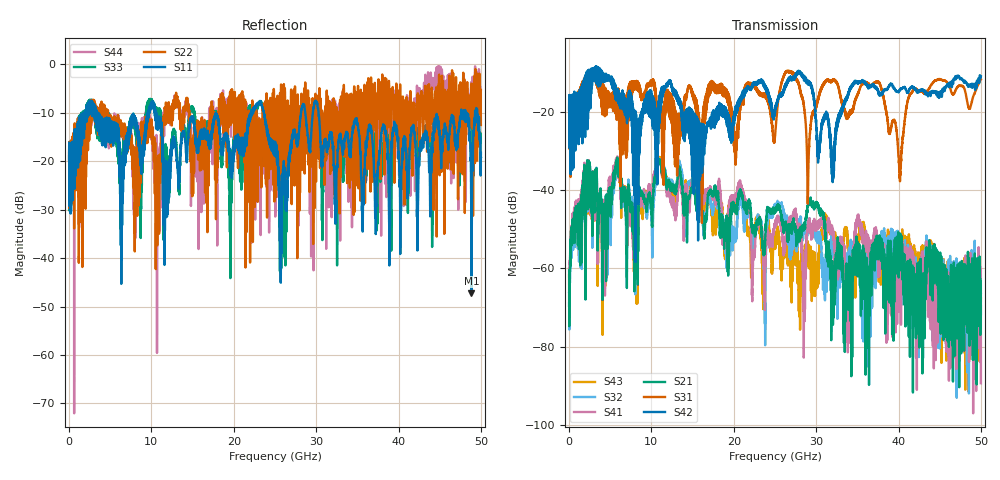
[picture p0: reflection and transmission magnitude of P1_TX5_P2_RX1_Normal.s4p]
!Keysight Technologies,N5225B,MY57041031,A.13.20.10
!Date: Friday, May 31, 2019 11:28:32
!Correction: S11(Full 4 Port(1,2,3,4))
!S12(Full 4 Port(1,2,3,4))
!S13(Full 4 Port(1,2,3,4))
!S14(Full 4 Port(1,2,3,4))
!S21(Full 4 Port(1,2,3,4))
!S22(Full 4 Port(1,2,3,4))
!S23(Full 4 Port(1,2,3,4))
!S24(Full 4 Port(1,2,3,4))
!S31(Full 4 Port(1,2,3,4))
!S32(Full 4 Port(1,2,3,4))
!S33(Full 4 Port(1,2,3,4))
!S34(Full 4 Port(1,2,3,4))
!S41(Full 4 Port(1,2,3,4))
!S42(Full 4 Port(1,2,3,4))
!S43(Full 4 Port(1,2,3,4))
!S44(Full 4 Port(1,2,3,4))
!S4P File: Measurements: <S11,S12,S13,S14>,
!<S21,S22,S23,S24>,
!<S31,S32,S33,S34>,
!<S41,S42,S43,S44>:
# Hz S  dB  R 50.0
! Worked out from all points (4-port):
!   5000 points, 10 MHz to 50 GHz, reference 50 ohm
!   strongest paths, dB at 10 MHz, 12.51 GHz, 25.01 GHz, 37.51 GHz, 50 GHz:
!     S42: -19.5, -14.3, -20.2, -14.6, -10.9
!     S31: -19.3, -23.1, -26.1, -12.2, -11.7
!     S21: -69.5, -38.9, -45.6, -55.1, -71.6
!     S41: -60.0, -42.5, -49.0, -56.1, -89.4
!     S32: -66.3, -37.4, -43.6, -53.9, -66.3
!     S43: -61.8, -40.2, -51.5, -57.7, -67.7
!   lowest |S11| = -47.3 dB at 48.86 GHz (marker M1), VSWR 1.01, Z = 50 - j0.434 ohm
!   |S11| at or under -10 dB: 3.502 GHz to 9.556 GHz (6.054 GHz wide, 92.7 % of centre); 10.5 GHz to 22.11 GHz (11.6 GHz wide, 71.2 % of centre); 30.29 GHz to 47.59 GHz (17.3 GHz wide, 44.4 % of centre)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
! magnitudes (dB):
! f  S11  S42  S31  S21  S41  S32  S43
! 10 MHz  -19.7  -19.5  -19.3  -69.5  -60.0  -66.3  -61.8
! 2.34 GHz  -8.8  -14.0  -12.0  -35.8  -35.7  -36.4  -36.7
! 8.13 GHz  -12.0  -23.2  -13.9  -46.4  -44.3  -52.0  -48.8
! 10.96 GHz  -12.9  -22.9  -19.0  -32.2  -32.2  -32.5  -31.8
! 25.8 GHz  -39.0  -15.7  -12.6  -46.2  -50.1  -43.4  -59.1
! 48.86 GHz  -47.3  -12.8  -17.7  -62.5  -67.3  -71.6  -66.8
! 50 GHz  -18.3  -10.9  -11.7  -71.6  -89.4  -66.3  -67.7
